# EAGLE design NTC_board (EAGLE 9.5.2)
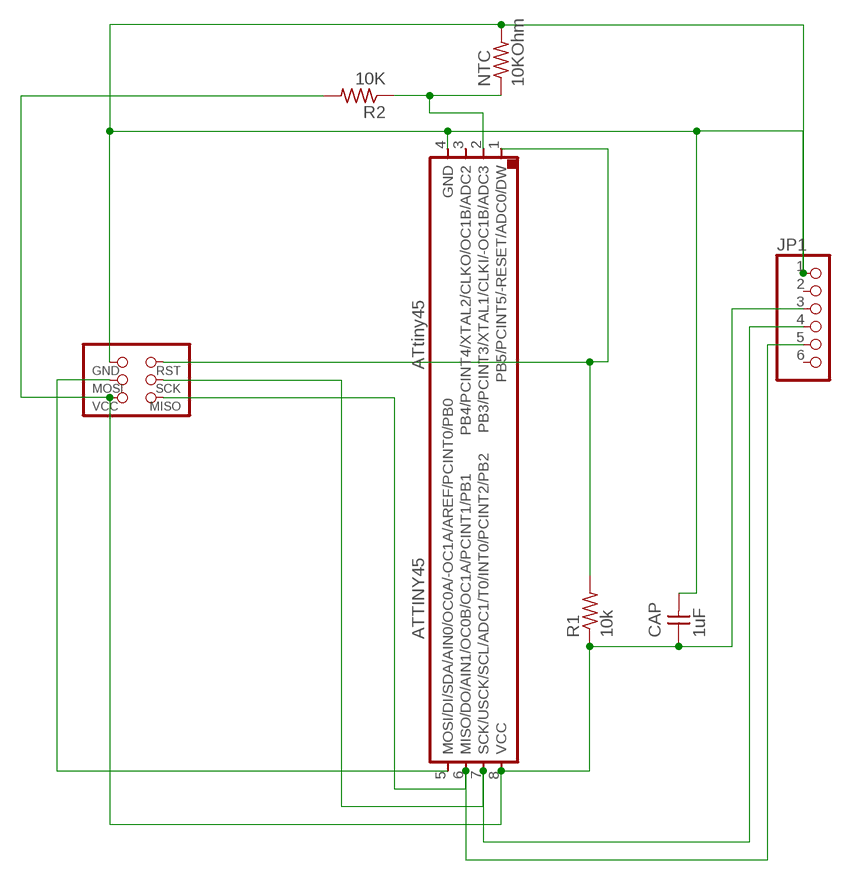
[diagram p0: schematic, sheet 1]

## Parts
ATTINY45  UC_ATTINY45SI  [SOIC8]
AVRISP  CONN_03X2_AVRISPSMD  [2X03SMD]
CAP  1uF  CAP_UNPOLARIZEDFAB  [C1206FAB]
JP1  PINHD-1X6  [1X06]
NTC  10KOhm  R1206FAB  [R1206FAB]
R1  10k  R1206FAB  [R1206FAB]
R2  10K  R1206FAB  [R1206FAB]

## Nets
AVRISP: ATTINY45.4(GND) AVRISP.6(GND) CAP.2 JP1.1 NTC.2
N$1: ATTINY45.2(PB3/PCINT3/XTAL1/CLKI/-OC1B/ADC3) NTC.1 R2.1
N$2: ATTINY45.5(MOSI/DI/SDA/AIN0/OC0A/-OC1A/AREF/PCINT0/PB0) AVRISP.4(MOSI)
N$3: ATTINY45.8(VCC) AVRISP.2(VCC) CAP.1 JP1.3 R1.1 R2.2
N$4: ATTINY45.6(MISO/DO/AIN1/OC0B/OC1A/PCINT1/PB1) AVRISP.1(MISO) JP1.5
N$6: ATTINY45.1(PB5/PCINT5/-RESET/ADC0/DW) AVRISP.5(RST) R1.2
N$8: ATTINY45.7(SCK/USCK/SCL/ADC1/T0/INT0/PCINT2/PB2) AVRISP.3(SCK) JP1.4
Unconnected: ATTINY45.3(PB4/PCINT4/XTAL2/CLKO/OC1B/ADC2) JP1.2 JP1.6

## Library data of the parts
ATTINY45 = fab:UC_ATTINY45
AVRISP = fab:CONN_03X2_AVRISP
CAP = fab:CAP_UNPOLARIZED
JP1 = pinhead:PINHD-1X6: PIN HEADER
NTC R1 R2 = fab:R: Resistor (US Symbol)

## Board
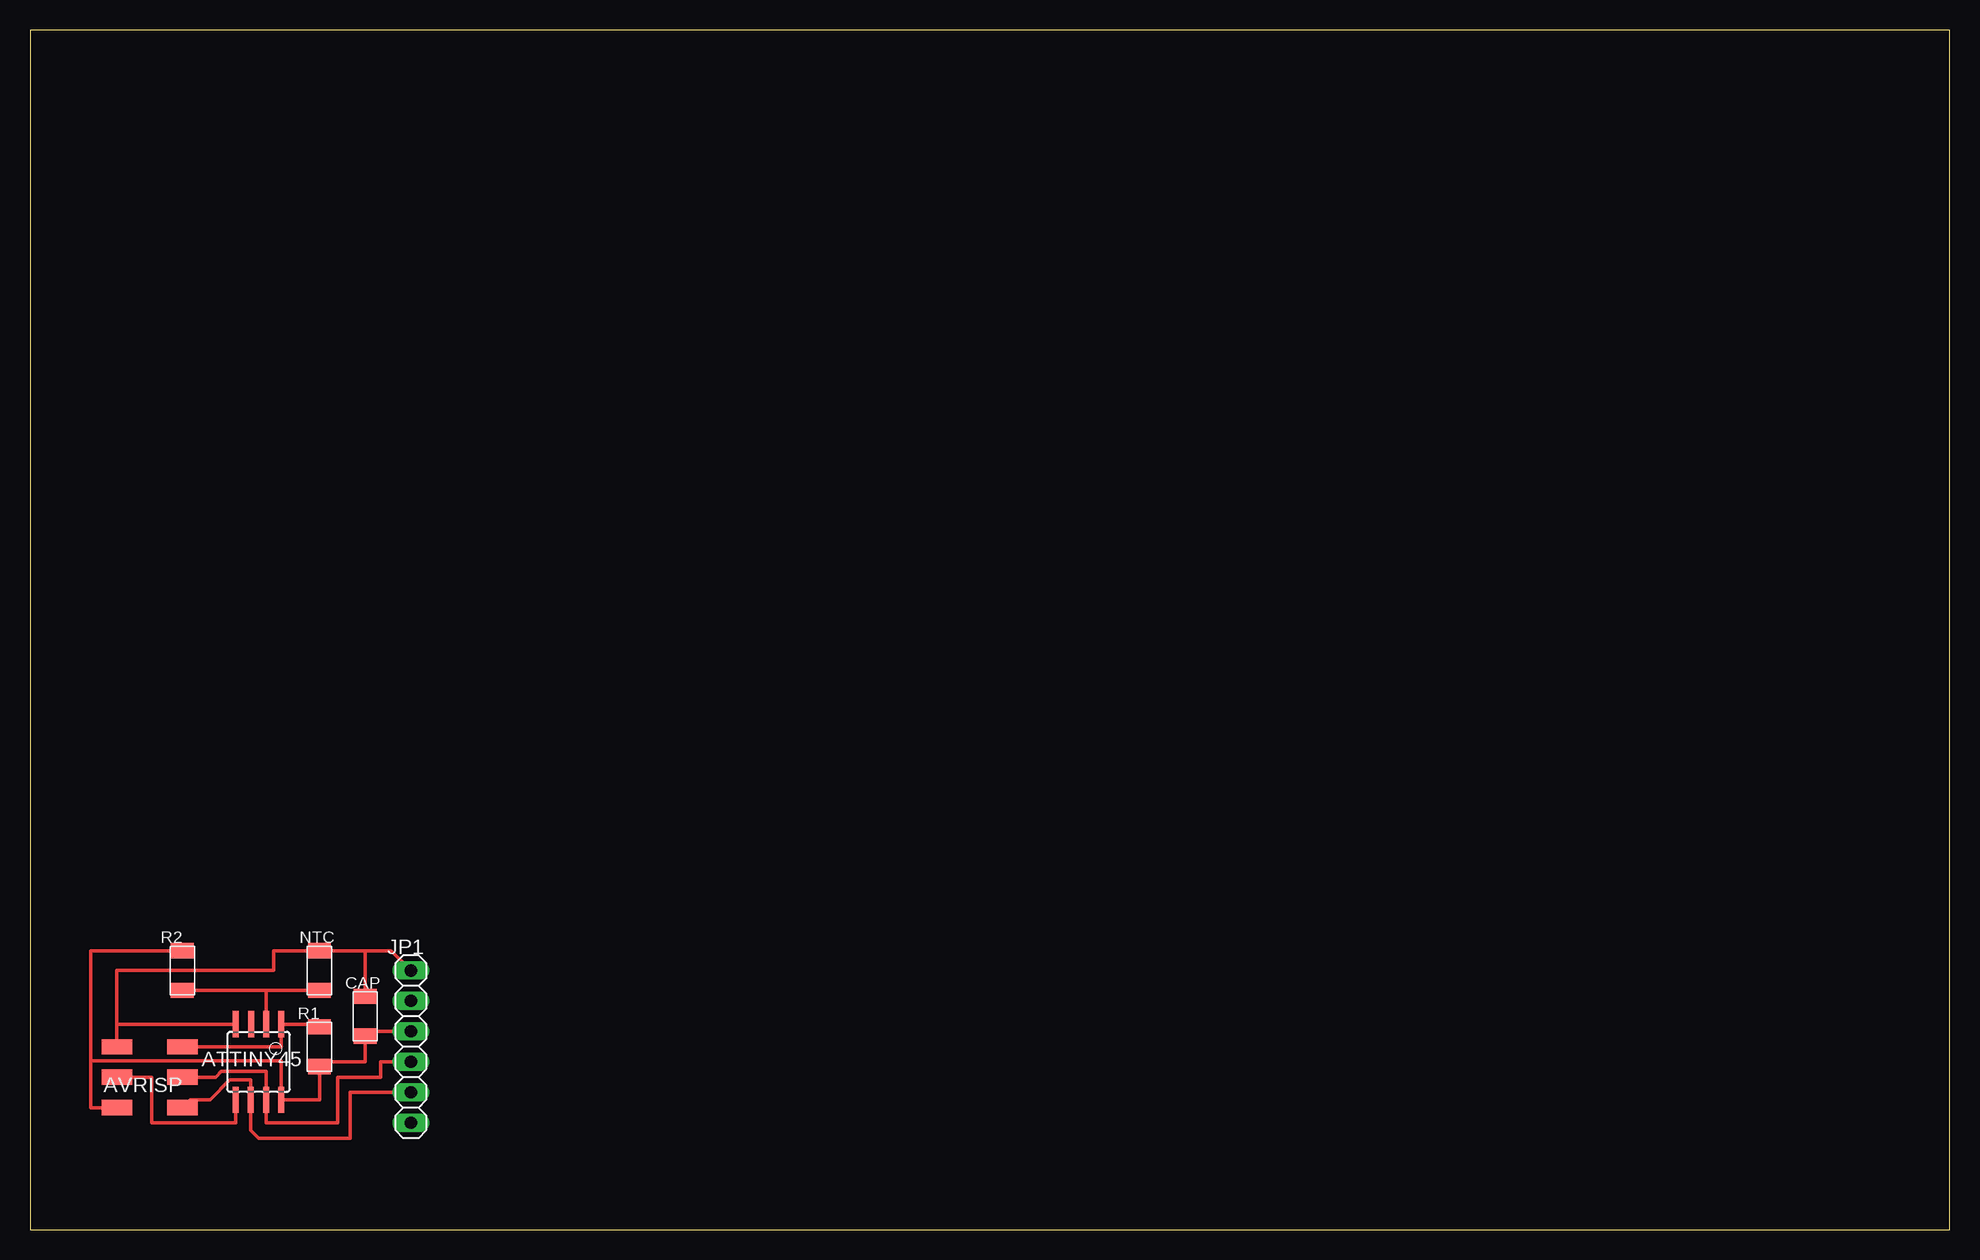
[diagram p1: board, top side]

Size 160 x 100 mm. Coordinates in mm from the lower left corner, seen from the top.
Outline: 0,0 160,0 160,100 0,100 0,0
Copper layers (1*16): Top 0.035mm / dielectric 1.5mm / Bottom 0.035mm
Design rules "default *": minimum track width 12mil, minimum drill 0.35mm, track to track 16mil, track to pad 16mil, pad to pad 16mil, via to via 16mil, smd to smd 16mil, copper to edge 16mil, drill to drill 16mil, minimum pad ring 10mil, minimum via ring 8mil, stop-mask expansion 4mil, vias tented up to drill 0mil, thermal gap 10mil

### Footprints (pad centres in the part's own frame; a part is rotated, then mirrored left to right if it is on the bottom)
SOIC8 = smd 0.5 x 2.2: 1 -1.905,-3.154; 2 -0.645,-3.154; 3 0.625,-3.154; 4 1.895,-3.154; 5 1.905,3.154; 6 0.635,3.154; 7 -0.635,3.154; 8 -1.905,3.154
2X03SMD = smd 2.54 x 1.27: 1 -2.54,2.54; 2 2.92,2.54; 3 -2.54,0; 4 2.92,0; 5 -2.54,-2.54; 6 2.92,-2.54
C1206FAB = smd 1.27 x 1.905: 1 -1.651,0; 2 1.651,0
1X06 = drill 1.016 long: 1 -6.35,0; 2 -3.81,0; 3 -1.27,0; 4 1.27,0; 5 3.81,0; 6 6.35,0
R1206FAB = smd 1.27 x 1.905: 1 -1.651,0; 2 1.651,0

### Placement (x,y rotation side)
ATTINY45  19.05,13.97 180 top
AVRISP  10.16,12.7 180 top
CAP  27.94,17.78 90 top
JP1  31.75,15.24 270 top
NTC  24.13,21.59 90 top
R1  24.13,15.24 90 top
R2  12.7,21.59 90 top

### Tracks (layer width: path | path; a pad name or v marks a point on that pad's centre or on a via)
AVRISP
  Top 0.305: 27.94,23.24 NTC.2 20.32,23.24 20.32,21.59 7.24,21.59 7.24,17.12 | 27.94,23.24 30.1,23.24 JP1.1 | CAP.2 27.94,23.24 | AVRISP.6 7.24,16.51 7.24,17.12 | ATTINY45.4 7.24,17.12
N$1
  Top 0.305: NTC.1 19.7,19.94 | 19.7,19.94 ATTINY45.2 | R2.1 19.7,19.94
N$2
  Top 0.305: AVRISP.4 10.16,12.7 10.16,8.89 17.14,8.89 ATTINY45.5
N$3
  Top 0.305: AVRISP.2 5.08,10.16 5.08,13.97 | 5.08,13.97 5.08,23.24 R2.2 | 5.08,13.97 5.16,14.05 20.95,14.05 ATTINY45.8 24.13,10.82 R1.1 24.13,13.97 27.94,13.97 CAP.1 27.94,16.51 JP1.3
N$4
  Top 0.305: AVRISP.1 13.36,10.82 15.01,10.82 16.66,12.47 18.41,12.47 ATTINY45.6 18.41,8.26 19.05,7.62 26.67,7.62 26.67,11.43 JP1.5
N$6
  Top 0.305: R1.2 24.13,17.12 ATTINY45.1 20.95,15.24 AVRISP.5
N$8
  Top 0.305: AVRISP.3 15.47,12.7 15.95,13.19 19.68,13.19 ATTINY45.7 19.68,8.89 25.64,8.89 25.64,12.7 29.21,12.7 29.21,13.97 JP1.4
